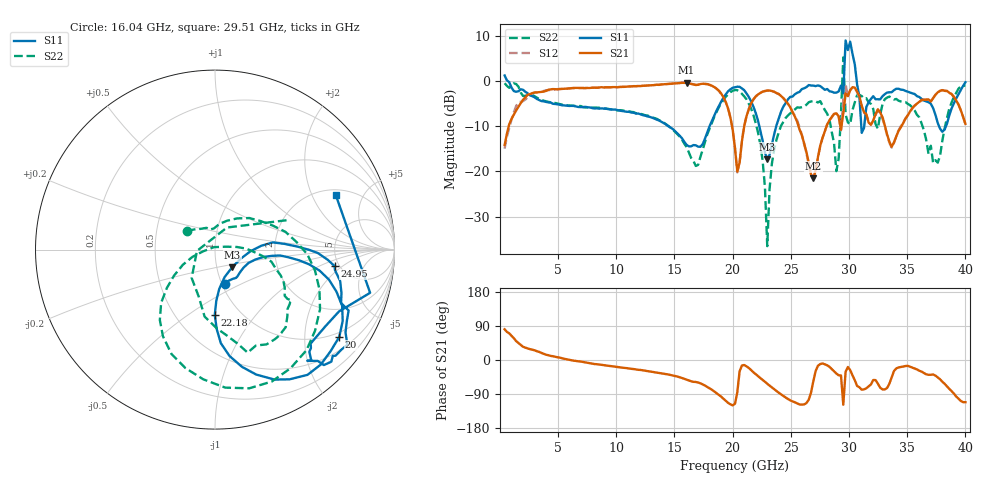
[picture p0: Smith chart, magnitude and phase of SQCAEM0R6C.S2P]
! Network Analyzer HP8722ES.07.66: Jul 25, 2000 Serial No. US39175408
! 26 Oct 2004  09:15:55
! Frequency  S11  S21  S12  S22
# HZ  S  DB R  50
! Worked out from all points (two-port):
!   201 points, 400 MHz to 40 GHz, reference 50 ohm
!   highest |S21| = -0.33 dB at 16.04 GHz (marker M1); lowest = -21.6 dB at 26.93 GHz (marker M2)
!   |S21| within 3 dB of the highest: 2.264 GHz to 19.16 GHz (16.9 GHz wide, 158 % of centre); 22 GHz to 24.19 GHz (2.188 GHz wide, 9.48 % of centre)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
!   lowest |S11| = -17.3 dB at 22.97 GHz (marker M3), VSWR 1.32, Z = 59.3 - j11.8 ohm
!   |S11| at or under -10 dB: 14.49 GHz to 18.01 GHz (3.519 GHz wide, 21.7 % of centre); 22.29 GHz to 23.74 GHz (1.448 GHz wide, 6.29 % of centre); 37.74 GHz to 38.32 GHz (581.8 MHz wide, 1.53 % of centre)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
!   |S22| runs from -36.6 to 5.3 dB; largest |S21 - S12| = 0.27
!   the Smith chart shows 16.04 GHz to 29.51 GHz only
!   S11 on the Smith chart (normalised r, x): 16.04 GHz: 1.03, -0.41; 20 GHz: 0.86, -2.94; 22.18 GHz: 0.76, -0.64; 24.95 GHz: 4.57, -1.53; 29.51 GHz: 2.31, +3.06
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4e8  1.29 -9.3  -14.15 81.1  -14.96 85.3  -0.43 -3.2
7.132e9  -5.75 -86.4  -1.49 -5.1  -1.51 -6.0  -5.71 -106.1
1.3666e10  -8.68 -91.7  -0.80 -34.2  -0.76 -34.1  -8.62 -156.6
1.6042e10  -14.10 -74.3  -0.33 -51.8  -0.33 -51.6  -14.60 146.9
2.0002e10  -1.45 -35.1  -10.75 -119.6  -10.76 -119.7  -2.12 -57.6
2.02e10  -1.34 -41.3  -14.84 -115.6  -14.79 -115.1  -1.94 -66.7
2.218e10  -8.76 -90.2  -2.92 -42.6  -2.89 -41.8  -11.38 -147.7
2.2972e10  -17.26 -45.6  -2.07 -62.6  -2.04 -61.7  -36.56 111.7
2.4952e10  -3.45 -7.8  -5.77 -106.4  -5.80 -105.5  -7.09 -28.6
2.6932e10  -0.97 -41.4  -21.55 -56.3  -21.72 -56.5  -4.43 -56.3
2.8912e10  -2.51 -34.9  -7.10 -35.8  -7.13 -36.0  -19.93 -175.8
2.9308e10  -0.94 -15.6  -10.75 -40.8  -10.87 -41.6  -7.15 22.0
2.9506e10  -2.64 24.1  -7.08 -118.0  -4.08 -99.3  5.32 57.1
2.9704e10  9.05 -26.7  -2.68 -31.1  -0.59 -18.8  -7.41 -81.0
3.01e10  8.77 -71.0  -1.95 -26.7  -2.01 -26.9  -9.56 -17.1
3.0496e10  3.72 -90.8  -1.40 -53.3  -1.53 -53.6  -4.69 -38.3
3.0694e10  -0.70 71.4  -2.28 -68.5  -2.41 -69.1  -3.10 130.2
3.1288e10  -10.34 133.1  -6.85 -77.5  -6.96 -78.7  -3.84 108.2
3.1486e10  -5.71 -37.9  -7.31 -74.6  -7.34 -76.2  -3.75 -77.4
3.3466e10  -2.44 -29.2  -13.41 -62.7  -13.65 -62.8  -3.39 -82.8
3.7624e10  -9.25 -78.6  -2.45 -45.9  -2.52 -46.2  -18.05 172.1
4e10  -0.22 -34.5  -9.44 -111.3  -9.59 -111.4  -0.95 -20.4
